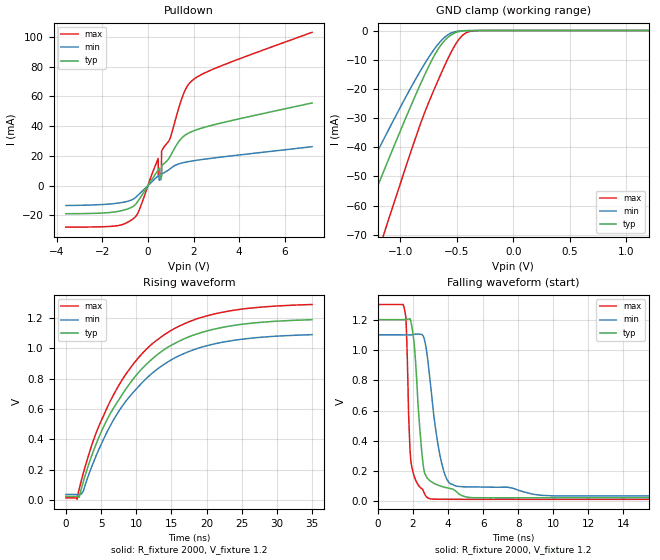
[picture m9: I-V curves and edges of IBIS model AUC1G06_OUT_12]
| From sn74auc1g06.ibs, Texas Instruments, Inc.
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[Model]   AUC1G06_OUT_12
Model_type  Open_drain
Enable   Active-Low
Vref =   0
Rref =   2000
Cref =   15p
Vmeas =   0.6
| variable   typ   min   max
C_comp   2.80pF   2.35pF   3.29pF
| C_pulldown   3.86pF   2.12pF   4.76pF
| C_tri-state   2.80pF   2.35pF   3.29pF
[Temperature Range]   40   100   -40
| Ambient temperature   25   85   -40
[Voltage range]   1.2   1.1   1.3
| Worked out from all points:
|   slope of the pulldown table from 0 to 0.18 V, typ, clamps not added: 42.4 ohm
|   GND clamp passes 1 mA (typ) near -0.53 V on its own axis
|   rising waveform, R_fixture 2000, V_fixture 1.2: 20-80 % time 9.53ns typ, 9.57ns min, 9.33ns max; typ from 0.024 V to 1.19 V
|   falling waveform, R_fixture 2000, V_fixture 1.2: 20-80 % time 443ps typ, 753ps min, 227ps max; typ from 1.2 V to 0.024 V
[GND Clamp]
| AUC1G06_OUT_12
|   Voltage   I(typ)   I(min)   I(max)
-3.6V     -288.1mA   -237.2mA   -357.2mA
-1.575V   -89.37mA   -70.5mA    -120.5mA
-1.525V   -84.5mA    -66.52mA   -114.6mA
-1.345V   -67.04mA   -52.36mA   -93.25mA
-1.14V    -47.42mA   -36.61mA   -68.88mA
-835mV    -19.39mA   -14.59mA   -33.3mA
-695mV    -8.236mA   -6.096mA   -19.61mA
-575mV    -2.185mA   -1.34mA    -9.275mA
-500mV    -555.7uA   -275.6uA   -4.012mA
-440mV    -130.5uA   -66.83uA   -1.345mA
-315mV    -3.46uA    -2.789uA   -28.94uA
1.2V      258.8pA    427.1pA    238.4pA
[Pulldown]
| AUC1G06_OUT_12
|   Voltage   I(typ)   I(min)   I(max)
-3.6V     -18.86mA   -13.33mA   -27.86mA
-1.33V    -17.35mA   -11.75mA   -26.87mA
-535mV    -12.4mA    -7.815mA   -20.65mA
450mV     10.5mA     6.398mA    18.24mA
455mV     10.61mA    6.451mA    6.435mA
590mV     5.848mA    7.731mA    8.546mA
600mV     5.947mA    7.818mA    22.94mA
605mV     12.96mA    7.861mA    23.36mA
970mV     19.55mA    11.32mA    31.69mA
1.615V    33.74mA    15.67mA    63.6mA
1.985V    36.72mA    16.71mA    71.17mA
7.2V      55.56mA    26.19mA    103mA
[Ramp]
| AUC1G06_OUT_12
| variable   typ   min   max
dV/dt_r   0.70/9.53E-09   0.63/9.58E-09   0.77/9.34E-09
dV/dt_f   0.71/4.60E-10   0.64/7.63E-10   0.77/2.44E-10
R_load = 2000
[Rising Waveform]
| AUC1G06_OUT_12
R_fixture =   2000
C_fixture =   0
L_fixture =   0
V_fixture =   1.2
V_fixture_min = 1.1
V_fixture_max = 1.3
|   Time   V(typ)   V(min)   V(max)
0s        23.98mV    36.64mV    13.86mV
1.59ns    23.92mV    36.53mV    4.672mV
1.88ns    18.37mV    36.69mV    69.82mV
2.5ns     123.8mV    60.93mV    180.1mV
3.975ns   329.8mV    254.5mV    401.1mV
6.41ns    577.3mV    497.7mV    661.2mV
9.35ns    784.6mV    698mV      882mV
12.57ns   942.1mV    847.6mV    1.041V
21.06ns   1.127V     1.029V     1.226V
34.99ns   1.189V     1.09V      1.289V
[Falling Waveform]
| AUC1G06_OUT_12
R_fixture =   2000
C_fixture =   0
L_fixture =   0
V_fixture =   1.2
V_fixture_min = 1.1
V_fixture_max = 1.3
|   Time   V(typ)   V(min)   V(max)
0s        1.2V       1.1V       1.3V
1.515ns   1.2V       1.1V       1.268V
1.615ns   1.201V     1.099V     1.161V
1.84ns    1.206V     1.099V     325mV
2.07ns    1.038V     1.103V     166.2mV
2.555ns   267.7mV    1.097V     78.29mV
2.905ns   142.7mV    870.9mV    19.58mV
3.625ns   99.17mV    257.2mV    14.35mV
4.455ns   67.15mV    101.5mV    13.9mV
34.99ns   23.98mV    36.64mV    13.86mV
